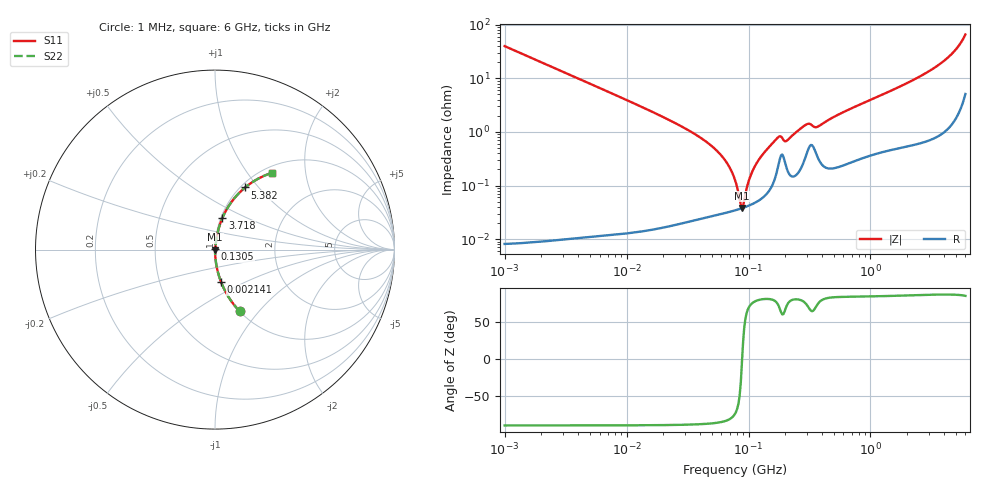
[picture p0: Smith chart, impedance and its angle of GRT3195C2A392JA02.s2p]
!Murata Part Number: GRT3195C2A392JA02
!These Parameters are Measured in Series Mode Connection
!Data Generated on Jun 19, 2026
!  o--ll--o
!Port1  Port2
!  o------o
!Operation Temp=25[degC], DC Bias Voltage=0[V]
!Freq. Start=1000[kHz] Stop=6[GHz] 401[Steps]
# Hz S RI R 50
!Freq.(Hz) S11(Real) S11(Imag) S21(Real) S21(Imag) S12(Real) S12(Imag) S22(Real) S22(Imag)
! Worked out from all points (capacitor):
!   401 points, 1 MHz to 6 GHz, reference 50 ohm
!   read as one part in series: C = 3.98 nF near 1.044 MHz
!   lowest |Z| = 38 mohm at 88.26 MHz (marker M1)
!   series resonance near 88.65 MHz, so ESL is about 810 pH
!   S11 on the Smith chart (normalised r, x): 1 MHz: 1.00, -0.80; 2.141 MHz: 1.00, -0.37; 130.5 MHz: 1.00, +0.01; 3.718 GHz: 1.02, +0.37; 5.382 GHz: 1.05, +0.85; 6 GHz: 1.10, +1.31
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1000000  0.1377 -0.3445  0.8623 0.3445  0.8623 0.3445  0.1377 -0.3445
2140860  0.0337 -0.1802  0.9663 0.1802  0.9663 0.1802  0.0337 -0.1802
4293785  0.00864 -0.092  0.9914 0.092  0.9914 0.092  0.00864 -0.092
1.843659e7  0.000586 -0.0207  0.9994 0.0207  0.9994 0.0207  0.000586 -0.0207
5.013812e7  0.000296 -0.0054  0.9997 0.0054  0.9997 0.0054  0.000296 -0.0054
6.508975e7  0.000317 -0.00282  0.9997 0.00282  0.9997 0.00282  0.000317 -0.00282
7.745967e7  0.000346 -0.00122  0.9997 0.00122  0.9997 0.00122  0.000346 -0.00122
8.450008e7  0.000366 -0.000434  0.9996 0.000434  0.9996 0.000434  0.000366 -0.000434
8.825674e7  0.000378 -3.98e-05  0.9996 3.98e-05  0.9996 3.98e-05  0.000378 -3.98e-05
9.218041e7  0.000391 0.000356  0.9996 -0.000356  0.9996 -0.000356  0.000391 0.000356
1.005588e8  0.000423 0.00116  0.9996 -0.00116  0.9996 -0.00116  0.000423 0.00116
1.073387e8  0.000454 0.00177  0.9995 -0.00177  0.9995 -0.00177  0.000454 0.00177
1.305463e8  0.000605 0.00374  0.9994 -0.00374  0.9994 -0.00374  0.000605 0.00374
1.770109e8  0.00262 0.00769  0.9974 -0.00769  0.9974 -0.00769  0.00262 0.00769
2.061188e8  0.00209 0.00652  0.9979 -0.00652  0.9979 -0.00652  0.00209 0.00652
2.919064e8  0.00345 0.0129  0.9966 -0.0129  0.9966 -0.0129  0.00345 0.0129
3.325952e8  0.00574 0.0118  0.9943 -0.0118  0.9943 -0.0118  0.00574 0.0118
3.708027e8  0.00341 0.0121  0.9966 -0.0121  0.9966 -0.0121  0.00341 0.0121
1.428092e9  0.00767 0.0561  0.9923 -0.0561  0.9923 -0.0561  0.00767 0.0561
3.718373e9  0.0412 0.1767  0.9588 -0.1767  0.9588 -0.1767  0.0412 0.1767
5.38176e9  0.1682 0.3464  0.8318 -0.3464  0.8318 -0.3464  0.1682 0.3464
6e9  0.3155 0.4274  0.6845 -0.4274  0.6845 -0.4274  0.3155 0.4274
